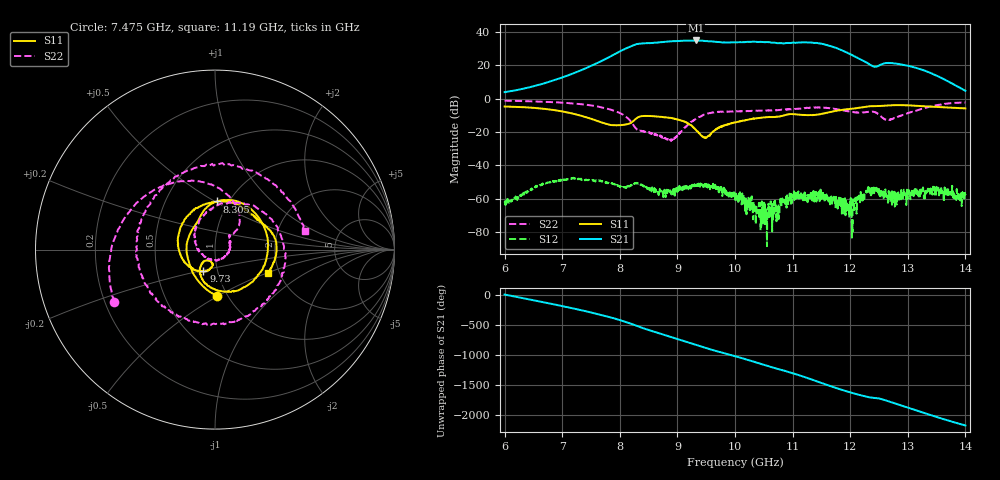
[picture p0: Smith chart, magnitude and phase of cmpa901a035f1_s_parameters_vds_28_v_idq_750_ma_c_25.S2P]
!Keysight Technologies,E5071C,MY46110325,B.14.03
!Date: Wed Mar 10 11:01:51 2021
!Data & Calibration Information:
!Freq	S11:SOLT2(ON)	S21:SOLT2(ON)	S12:SOLT2(ON)	S22:SOLT2(ON)
!PortZ  Port1:50+j0  Port2:50+j0
!Above PortZ is port z conversion or system Z0 setting when saving the data.
!When reading, reference impedance value at option line is always used.
# Hz S dB R 50
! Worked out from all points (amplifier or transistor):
!   1601 points, 6 GHz to 14 GHz, reference 50 ohm
!   highest |S21| = 34.7 dB at 9.32 GHz (marker M1)
!   |S21| within 3 dB of that: 8.23 GHz to 11.62 GHz (3.39 GHz wide, 34.2 % of centre)
!   unconditionally stable (mu >= 1): start of sweep to end of sweep
!   at 7.33 GHz: K = 9.27, MAG = 20.0 dB, |S12| = -48.3 dB
!   at 10 GHz: K = 7.01, MAG = 34.6 dB, |S12| = -58.4 dB
!   at 14 GHz: K = 69.06, MAG = 9.8 dB, |S12| = -57.7 dB
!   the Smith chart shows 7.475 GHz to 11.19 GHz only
!   S11 on the Smith chart (normalised r, x): 7.475 GHz: 0.90, -0.49; 8.305 GHz: 0.88, +0.51; 9.73 GHz: 0.85, -0.21; 11.19 GHz: 1.75, -0.51
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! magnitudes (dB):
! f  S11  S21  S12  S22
! 6 GHz  -4.7  3.8  -62.3  -1.3
! 6.7 GHz  -6.2  9.2  -50.8  -2.0
! 7.335 GHz  -10.3  17.1  -48.3  -3.4
! 7.475 GHz  -11.8  19.1  -48.8  -4.0
! 8.01 GHz  -15.9  28.3  -52.5  -8.8
! 8.305 GHz  -11.4  32.6  -50.6  -18.7
! 8.67 GHz  -10.8  33.6  -57.0  -21.7
! 8.925 GHz  -11.8  34.3  -57.3  -24.0
! 9.32 GHz  -18.6  34.7  -51.5  -12.2
! 9.485 GHz  -23.3  34.4  -51.4  -9.5
! 9.73 GHz  -17.3  33.7  -53.5  -7.9
! 10 GHz  -14.3  33.6  -58.4  -7.7
! 10.56 GHz  -11.0  33.7  -69.3  -7.1
! 10.82 GHz  -10.4  33.0  -59.7  -6.7
! 11.19 GHz  -9.8  33.7  -60.8  -5.8
! 11.34 GHz  -9.9  33.4  -56.5  -5.4
! 11.7 GHz  -7.7  30.9  -58.5  -6.1
! 12 GHz  -6.2  26.5  -67.9  -7.8
! 12.29 GHz  -4.8  21.3  -56.3  -8.1
! 12.67 GHz  -4.1  21.3  -55.2  -12.9
! 13.47 GHz  -4.9  14.1  -53.4  -4.2
! 14 GHz  -5.9  4.6  -57.7  -2.3
